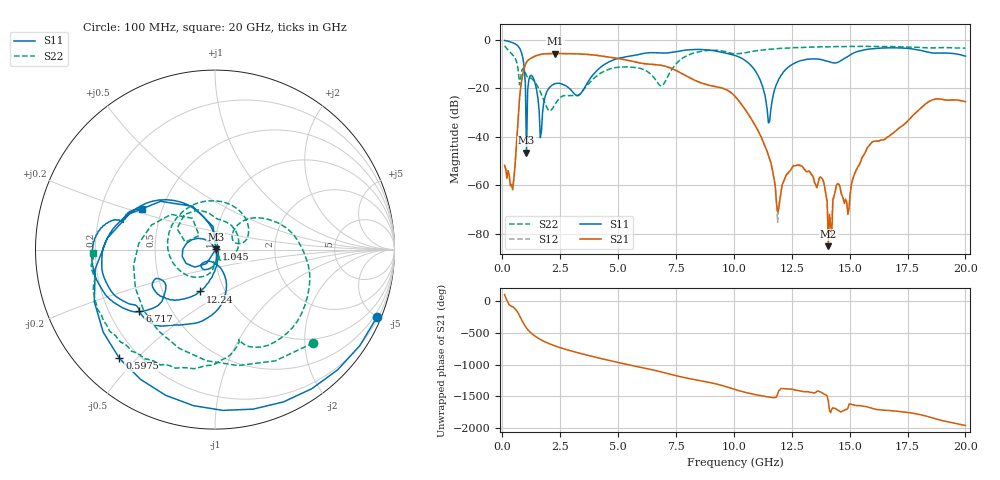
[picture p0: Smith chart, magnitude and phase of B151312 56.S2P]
!  2-Port S-parameters saved by WinCal
! VAR MeasName=S-Parameters (CALIBRATED_DATA) read from VNA (N5244A)
! VAR MeasDate=12/8/2015 5:48:09 PM
! VAR NAME=B151312 56
! VAR FILENAME=B151312 56.S2P
! VAR DATE=12/8/2015 5:48:09 PM
! VAR PHYS_PORTS=1,2
# Hz S DB R 50
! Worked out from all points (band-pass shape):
!   401 points, 100 MHz to 20 GHz, reference 50 ohm
!   highest |S21| = -5.59 dB at 2.289 GHz (marker M1); lowest = -85.2 dB at 14.08 GHz (marker M2)
!   |S21| within 3 dB of the highest: 1.092 GHz to 5.51 GHz (4.418 GHz wide, 134 % of centre)
!   lowest |S11| = -46.5 dB at 1.045 GHz (marker M3), VSWR 1.01, Z = 50.4 + j0.167 ohm
!   |S11| at or under -10 dB: 926.8 MHz to 4.428 GHz (3.502 GHz wide, 131 % of centre); 10.69 GHz to 12.54 GHz (1.851 GHz wide, 15.9 % of centre)
!   |S22| runs from -29.2 to -2.4 dB; largest |S21 - S12| = 0.0017
!   S11 on the Smith chart (normalised r, x): 100 MHz: 0.29, -4.99; 597.5 MHz: 0.13, -0.45; 1.045 GHz: 1.01, +0.00; 6.717 GHz: 0.33, -0.32; 12.24 GHz: 0.77, -0.38; 20 GHz: 0.39, +0.22
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1e8  -0.20 -22.6  -51.74 97.9  -51.98 96.7  -2.44 -43.5
4.4825e8  -1.13 -97.9  -61.88 -91.0  -60.75 -93.3  -6.15 -154.2
5.975e8  -1.86 -131.3  -45.13 -146.0  -45.10 -146.3  -8.42 158.8
7.965e8  -4.37 174.1  -19.35 87.7  -19.35 87.7  -15.37 166.0
1.04525e9  -46.52 20.5  -9.19 -66.5  -9.20 -66.5  -14.73 91.9
1.44325e9  -18.86 146.6  -6.56 158.8  -6.56 158.8  -17.86 3.1
1.692e9  -37.72 -63.2  -5.90 104.3  -5.90 104.3  -22.53 -54.9
2.289e9  -18.01 -117.6  -5.59 11.2  -5.60 11.2  -26.49 -61.1
3.43325e9  -21.57 -83.9  -5.81 -110.9  -5.81 -110.9  -21.49 -94.4
5.075e9  -7.46 -104.9  -7.74 106.9  -7.74 107.0  -11.18 150.0
6.71675e9  -5.30 -140.8  -10.27 -22.0  -10.27 -22.2  -17.80 15.5
6.7665e9  -5.32 -141.4  -10.33 -26.5  -10.33 -26.6  -18.42 18.0
1.005e10  -6.39 149.3  -23.28 48.9  -23.29 48.6  -5.69 -75.2
1.099525e10  -13.83 110.6  -36.58 -35.9  -36.59 -36.2  -4.42 -83.1
1.149275e10  -34.28 35.9  -47.58 -67.1  -47.62 -67.7  -3.84 -91.2
1.189075e10  -17.30 -94.4  -71.02 -19.0  -75.34 -6.9  -3.55 -98.0
1.2239e10  -12.13 -109.4  -56.32 62.0  -56.34 59.6  -3.39 -102.5
1.338325e10  -7.82 -144.7  -55.84 4.0  -55.79 2.6  -2.99 -117.7
1.3831e10  -8.29 -152.8  -57.51 -7.5  -57.64 -8.6  -2.82 -123.2
1.407975e10  -8.84 -153.6  -85.18 -133.3  -79.49 -90.8  -2.83 -126.4
1.67165e10  -3.27 -172.1  -39.67 79.4  -39.65 78.9  -2.69 -152.9
2e10  -6.68 151.0  -25.51 -154.5  -25.63 -154.9  -3.37 -178.5
